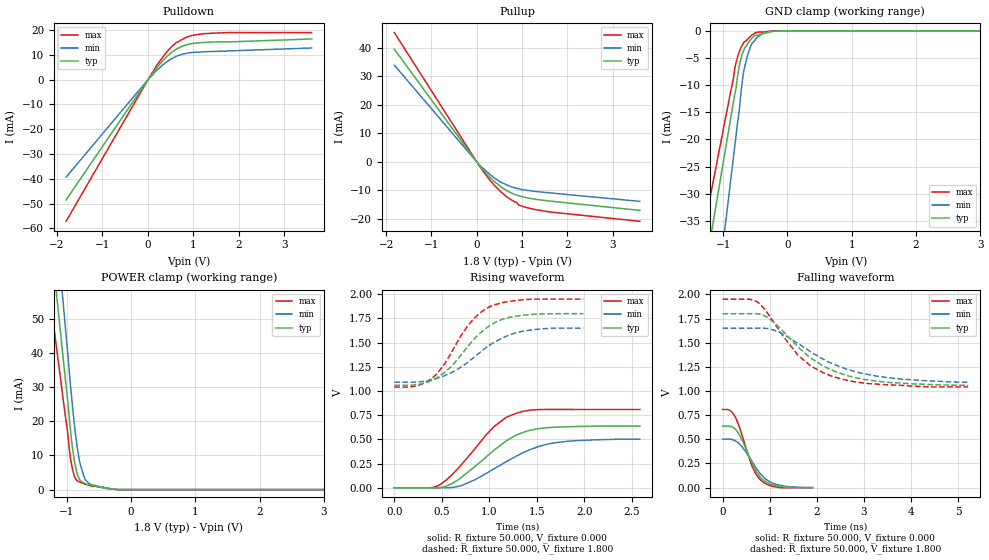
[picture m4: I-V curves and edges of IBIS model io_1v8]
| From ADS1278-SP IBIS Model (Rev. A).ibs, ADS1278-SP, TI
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[Model]   io_1v8
Model_type I/O
Vinl=5.400E-01
Vinh=1.260E+00
Vref=0.000E+00
Rref=1.000E+06
Cref=2.000E-11
Vmeas=9.000E-01
C_comp   698.00E-15   698.00E-15   698.00E-15
[Voltage Range]   1.800E+00   1.650E+00   1.950E+00
[POWER Clamp Reference]   1.800E+00   1.650E+00   1.950E+00
[GND Clamp Reference]   0.000E+00   0.000E+00   0.000E+00
[Pullup Reference]   1.800E+00   1.650E+00   1.950E+00
[Pulldown Reference]   0.000E+00   0.000E+00   0.000E+00
[Temperature Range]   25   105   -40
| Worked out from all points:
|   slope of the pulldown table from 0 to 0.27 V, typ, clamps not added: 41.6 ohm
|   slope of the pullup table from 0 to 0.27 V, typ, clamps not added: 53 ohm
|   GND clamp passes 1 mA (typ) near -0.52 V on its own axis
|   POWER clamp passes 1 mA (typ) near -0.51 V on its own axis
|   rising waveform, R_fixture 50.000, V_fixture 0.000: 20-80 % time 489ps typ, 570ps min, 436ps max; typ from 0 V to 0.637 V
|   falling waveform, R_fixture 50.000, V_fixture 0.000: 20-80 % time 373ps typ, 440ps min, 343ps max; typ from 0.637 V to 0 V
|   rising waveform, R_fixture 50.000, V_fixture 1.800: 20-80 % time 422ps typ, 490ps min, 375ps max; typ from 1.06 V to 1.8 V
|   falling waveform, R_fixture 50.000, V_fixture 1.800: 20-80 % time 1.15ns typ, 1.34ns min, 998ps max; typ from 1.8 V to 1.06 V
[GND Clamp]
-1.8V     -80.56mA   -118.8mA   -67.47mA
-1.76V    -77.75mA   -114.5mA   -64.75mA
-880mV    -15.9mA    -27.24mA   -10.98mA
-780mV    -8.706mA   -17.27mA   -4.994mA
-740mV    -5.894mA   -13.52mA   -3.569mA
-720mV    -4.964mA   -11.01mA   -2.964mA
-680mV    -3.562mA   -7.437mA   -2.148mA
-600mV    -2.04mA    -3.712mA   -1.299mA
-500mV    -856.2uA   -1.574mA   -387.6uA
-380mV    -462.2uA   -524.2uA   -234.2uA
-80mV     0A         0A         0A
3.6V      0A         0A         0A
[Power Clamp]
-1.82V    177.7mA    210.8mA    134.6mA
-1.76V    166.7mA    203mA      129.4mA
-1.04V    35.84mA    51.64mA    24.36mA
-980mV    25.34mA    39.15mA    15.89mA
-940mV    17.19mA    30.39mA    9.045mA
-920mV    13.76mA    26.46mA    6.924mA
-860mV    6.405mA    15.77mA    3.113mA
-820mV    3.704mA    10.48mA    2.384mA
-780mV    2.473mA    6.844mA    2.077mA
-700mV    1.652mA    2.657mA    1.529mA
-360mV    399.9uA    246.7uA    393.6uA
3.6V      0A         0A         0A
[Pullup]
-1.82V    39.55mA    33.95mA    45.39mA
100mV     -2.03mA    -1.693mA   -2.367mA
260mV     -4.94mA    -3.983mA   -5.808mA
400mV     -7.026mA   -5.742mA   -8.463mA
660mV     -10.08mA   -8.076mA   -12.21mA
880mV     -11.63mA   -9.258mA   -14.24mA
920mV     -11.84mA   -9.412mA   -15.09mA
1.22V     -12.91mA   -10.2mA    -16.49mA
1.6V      -13.71mA   -10.84mA   -17.54mA
3.6V      -17.01mA   -13.84mA   -20.83mA
[Pulldown]
-1.8V     -48.54mA   -39.33mA   -57.18mA
20mV      542.4uA    428.8uA    629uA
200mV     5.029mA    3.963mA    5.971mA
360mV     8.339mA    6.488mA    9.965mA
460mV     10.12mA    7.822mA    12.16mA
620mV     12.33mA    9.435mA    15mA
780mV     13.71mA    10.4mA     16.57mA
920mV     14.43mA    10.87mA    17.64mA
1.26V     15.06mA    11.3mA     18.62mA
1.78V     15.26mA    11.63mA    19.04mA
3.6V      16.46mA    12.82mA    19.04mA
[Rising Waveform]
R_fixture = 50.000
V_fixture = 0.000
V_fixture_min = 0.000
V_fixture_max = 0.000
|  time   V(typ)   V(min)   V(max)
0s        0V         0V         0V
385ps     -318.6uV   0V         1.501mV
490ps     4.296mV    -398uV     38.82mV
710ps     110.8mV    24.75mV    243.6mV
1.05ns    389.9mV    196.7mV    633.3mV
1.165ns   475.6mV    262.2mV    719.4mV
1.285ns   545.3mV    327.4mV    771mV
1.52ns    611.5mV    426.8mV    808.1mV
1.725ns   627.6mV    470.2mV    809.8mV
2.585ns   637.2mV    502.1mV    809.3mV
[Falling Waveform]
R_fixture = 50.000
V_fixture = 0.000
V_fixture_min = 0.000
V_fixture_max = 0.000
|  time   V(typ)   V(min)   V(max)
0s        637.2mV    502.1mV    809.3mV
145ps     637mV      502mV      800.9mV
265ps     607.9mV    486.9mV    735mV
430ps     478mV      413.6mV    518.1mV
615ps     267.5mV    279.3mV    234.7mV
720ps     162.3mV    197.9mV    132.3mV
835ps     90.89mV    126.2mV    66.45mV
975ps     44.68mV    68.05mV    27.33mV
1.185ns   13.75mV    27.81mV    2.642mV
1.91ns    0V         0V         0V
[Rising Waveform]
R_fixture = 50.000
V_fixture = 1.800
V_fixture_min = 1.650
V_fixture_max = 1.950
|  time   V(typ)   V(min)   V(max)
0s        1.06V      1.092V     1.043V
240ps     1.066V     1.094V     1.055V
405ps     1.115V     1.118V     1.14V
525ps     1.189V     1.157V     1.274V
600ps     1.254V     1.19V      1.397V
770ps     1.457V     1.295V     1.67V
875ps     1.572V     1.378V     1.784V
1.02ns    1.686V     1.485V     1.879V
1.36ns    1.784V     1.62V      1.944V
1.99ns    1.8V       1.65V      1.95V
[Falling Waveform]
R_fixture = 50.000
V_fixture = 1.800
V_fixture_min = 1.650
V_fixture_max = 1.950
|  time   V(typ)   V(min)   V(max)
0s        1.8V       1.65V      1.95V
725ps     1.799V     1.65V      1.926V
955ps     1.763V     1.646V     1.806V
1.29ns    1.615V     1.588V     1.565V
1.595ns   1.461V     1.495V     1.375V
1.89ns    1.335V     1.399V     1.255V
2.275ns   1.225V     1.295V     1.161V
2.855ns   1.135V     1.195V     1.092V
3.48ns    1.092V     1.14V      1.065V
5.215ns   1.06V      1.092V     1.043V
[Ramp]
dV/dt_r   3.720E-01/4.865E-10   3.027E-01/5.696E-10   4.853E-01/4.324E-10
dV/dt_f   4.440E-01/1.128E-09   3.346E-01/1.345E-09   5.445E-01/9.823E-10
R_load = 50
